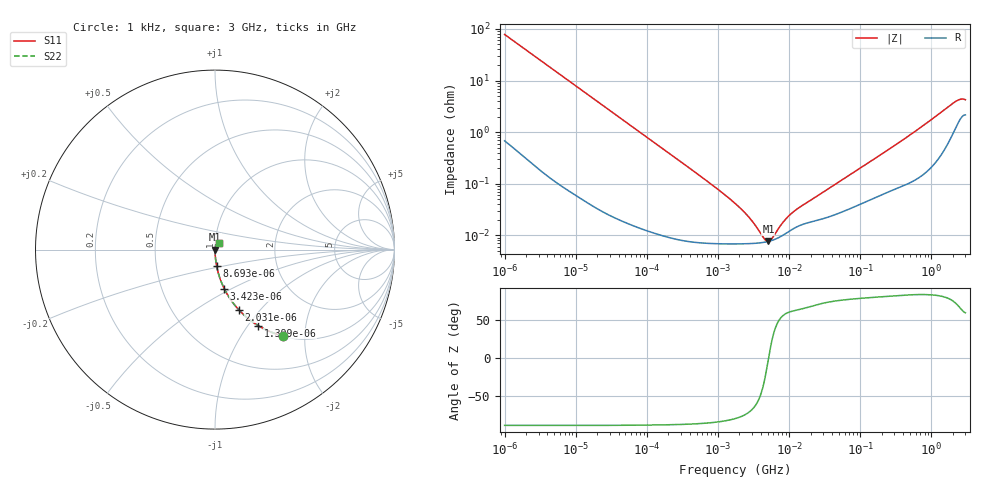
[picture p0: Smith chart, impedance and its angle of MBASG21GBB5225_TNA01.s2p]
! MBASG21GBB5225_TNA01  S-PARAMETER MODEL  ( Standard Model )
! Model Generated by TAIYO YUDEN Corporation (http://www.ty-top.com)
! Version 1.0
! TAIYO YUDEN Control No. 220601
! Copyright(c) 2014 TAIYO YUDEN CO.,LTD. All Rights Reserved.
! Product Description (link to TY-COMPAS)
! https://ds.yuden.co.jp/TYCOMPAS/or/detail?pn=MBASG21GBB5225KTNA01&u=M
! Products Name : Multilayer Ceramic Capacitors
! Characteristics :
!  Capacitance : 2.2 [uF] , Rated Voltage : 35 [V] , TCC : X5R
!  Case Size : 2.0 x 1.25 / 0.079 x 0.049 [mm/inch] , Thickness : 1.25 / 0.049 [mm/inch]
!  (Conditions: Temperature = 25 [degC] , DC Bias Voltage = 0 [V])
! External Node Assignments :
!  1  o---| |---o  2
! GND o---------o GND
! Frequency Range : 1kHz  -  3GHz  [ 401 STEP ]
# MHZ S RI R 50
! Freq[MHz].  S11 Real  S11 Imag  S21 Real  S21 Imag  S12 Real  S12 Imag  S22 Real  S22 Imag
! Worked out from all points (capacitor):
!   401 points, 1 kHz to 3 GHz, reference 50 ohm
!   read as one part in series: C = 2.03 uF near 1.077 kHz
!   lowest |Z| = 7.64 mohm at 5.107 MHz (marker M1)
!   series resonance near 5.144 MHz, so ESL is about 470 pH
!   S11 on the Smith chart (normalised r, x): 1 kHz: 1.01, -1.56; 1.399 kHz: 1.01, -1.12; 2.031 kHz: 1.01, -0.77; 3.423 kHz: 1.00, -0.46; 8.693 kHz: 1.00, -0.18; 3 GHz: 1.04, +0.07
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0.001  0.3799 -0.481  0.6201 0.481  0.6201 0.481  0.3799 -0.481
0.001399  0.2403 -0.4231  0.7597 0.4231  0.7597 0.4231  0.2403 -0.4231
0.002031  0.1317 -0.3343  0.8683 0.3343  0.8683 0.3343  0.1317 -0.3343
0.003423  0.0515 -0.2174  0.9485 0.2174  0.9485 0.2174  0.0515 -0.2174
0.008693  0.00882 -0.0899  0.9912 0.0899  0.9912 0.0899  0.00882 -0.0899
0.01216  0.0047 -0.0646  0.9953 0.0646  0.9953 0.0646  0.0047 -0.0646
0.033275  0.000794 -0.0238  0.9992 0.0238  0.9992 0.0238  0.000794 -0.0238
0.147855  0.000132 -0.0054  0.9999 0.0054  0.9999 0.0054  0.000132 -0.0054
0.762639  7.08e-05 -0.00103  0.9999 0.00103  0.9999 0.00103  7.08e-05 -0.00103
1.732051  6.84e-05 -0.000412  0.9999 0.000412  0.9999 0.000412  6.84e-05 -0.000412
2.709407  6.91e-05 -0.000215  0.9999 0.000215  0.9999 0.000215  6.91e-05 -0.000215
4.083148  7.22e-05 -7.35e-05  0.9999 7.35e-05  0.9999 7.35e-05  7.22e-05 -7.35e-05
4.399271  7.33e-05 -4.95e-05  0.9999 4.95e-05  0.9999 4.95e-05  7.33e-05 -4.95e-05
5.106836  7.63e-05 -2.26e-06  0.9999 2.26e-06  0.9999 2.26e-06  7.63e-05 -2.26e-06
6.153411  8.27e-05 5.67e-05  0.9999 -5.67e-05  0.9999 -5.67e-05  8.27e-05 5.67e-05
8.291982  0.000102 0.000152  0.9999 -0.000152  0.9999 -0.000152  0.000102 0.000152
10.37087  0.000124 0.000222  0.9999 -0.000222  0.9999 -0.000222  0.000124 0.000222
21.06097  0.000185 0.000466  0.9998 -0.000466  0.9998 -0.000466  0.000185 0.000466
256.0921  0.000727 0.00465  0.9993 -0.00465  0.9993 -0.00465  0.000727 0.00465
2066.299  0.0113 0.0352  0.9887 -0.0352  0.9887 -0.0352  0.0113 0.0352
2489.759  0.0182 0.0381  0.9818 -0.0381  0.9818 -0.0381  0.0182 0.0381
3000  0.0224 0.0351  0.9776 -0.0351  0.9776 -0.0351  0.0224 0.0351
